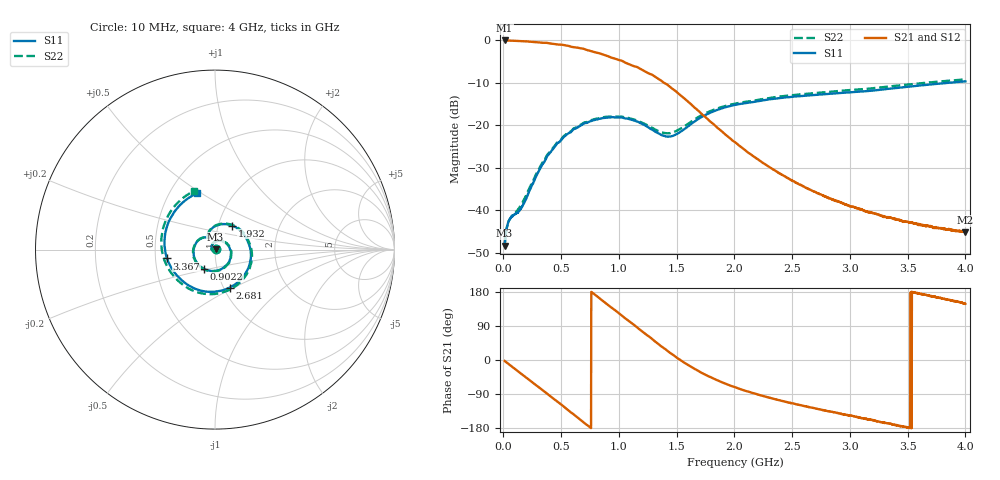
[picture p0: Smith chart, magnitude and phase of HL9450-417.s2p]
! 7/30/2020 11:09:13 AM
! H:\PROTOTYPE_DATA\9450\10029\HL9450_10013_840MHZ_.S2P
! CHANNEL.1
! TR.MEASUREMENT
! CORRECTED.DATA
# GHZ S RI R 50.0
! FREQ.GHZ  S11RE  S11IM  S21RE  S21IM  S12RE  S12IM  S22RE  S22IM
!; PortSelection: Port_12
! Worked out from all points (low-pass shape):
!   2000 points, 10 MHz to 4 GHz, reference 50 ohm
!   highest |S21| = -0.03 dB at 10 MHz (marker M1); lowest = -45.1 dB at 3.994 GHz (marker M2)
!   |S21| within 3 dB of the highest: start of sweep to 828.3 MHz
!   lowest |S11| = -48.3 dB at 10 MHz (marker M3), VSWR 1.01, Z = 50.4 + j0.154 ohm
!   |S11| at or under -10 dB: start of sweep to 3.847 GHz
!   |S22| runs from -48.4 to -9.2 dB; largest |S21 - S12| = 0.0061
!   S11 on the Smith chart (normalised r, x): 10 MHz: 1.01, +0.00; 902.2 MHz: 0.86, -0.19; 1.932 GHz: 1.16, +0.32; 2.681 GHz: 1.07, -0.48; 3.367 GHz: 0.58, -0.06; 4 GHz: 0.68, +0.48
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0.01  0.00351 0.00153  0.9956 -0.0426  0.9965 -0.0431  0.00349 0.00149
0.05391196  0.00762 -0.00179  0.967 -0.2211  0.9676 -0.221  0.0076 -0.00215
0.2036118  -0.0136 -0.00455  0.649 -0.7212  0.6487 -0.7209  -0.0149 -0.00492
0.3573037  -0.00775 0.0375  0.1028 -0.9281  0.1016 -0.928  -0.00902 0.0384
0.5050075  0.0558 0.0393  -0.4253 -0.779  -0.4258 -0.7792  0.0568 0.0414
0.6766633  0.0823 -0.0585  -0.7532 -0.2762  -0.7541 -0.2749  0.0847 -0.0583
0.7864432  0.0243 -0.1132  -0.7233 0.0802  -0.7252 0.0798  0.0265 -0.115
0.9022111  -0.0625 -0.1064  -0.541 0.3659  -0.5424 0.3649  -0.0612 -0.1104
1.109795  -0.1152 0.0158  -0.0664 0.5053  -0.0684 0.5056  -0.1186 0.0119
1.341331  -0.0443 0.067  0.2615 0.2383  0.2622 0.2357  -0.0507 0.0693
1.59083  -0.0365 0.0882  0.1893 -0.0393  0.1894 -0.0397  -0.0357 0.096
1.932146  0.096 0.1338  0.0337 -0.0681  0.0335 -0.0683  0.1058 0.1338
2.005998  0.1315 0.1142  0.0197 -0.0601  0.0193 -0.0601  0.1414 0.1113
2.337334  0.1992 -0.05  -0.00654 -0.0296  -0.00637 -0.0294  0.2041 -0.0616
2.670665  0.0862 -0.2091  -0.00997 -0.0138  -0.00997 -0.0138  0.0821 -0.2234
2.680645  0.0808 -0.2119  -0.00994 -0.0136  -0.01 -0.0136  0.0763 -0.226
2.980045  -0.1025 -0.2213  -0.00941 -0.00647  -0.00944 -0.00646  -0.1145 -0.2321
3.335333  -0.26 -0.0687  -0.00806 -0.00181  -0.00806 -0.00184  -0.277 -0.0716
3.367269  -0.2673 -0.049  -0.00796 -0.00135  -0.00793 -0.00148  -0.2847 -0.0509
3.664672  -0.2606 0.1477  -0.0066 0.000984  -0.00649 0.000924  -0.2773 0.154
3.994012  -0.1063 0.311  -0.00477 0.00281  -0.00489 0.00295  -0.119 0.3259
4  -0.1031 0.313  -0.00476 0.00293  -0.0048 0.0028  -0.1149 0.3274
